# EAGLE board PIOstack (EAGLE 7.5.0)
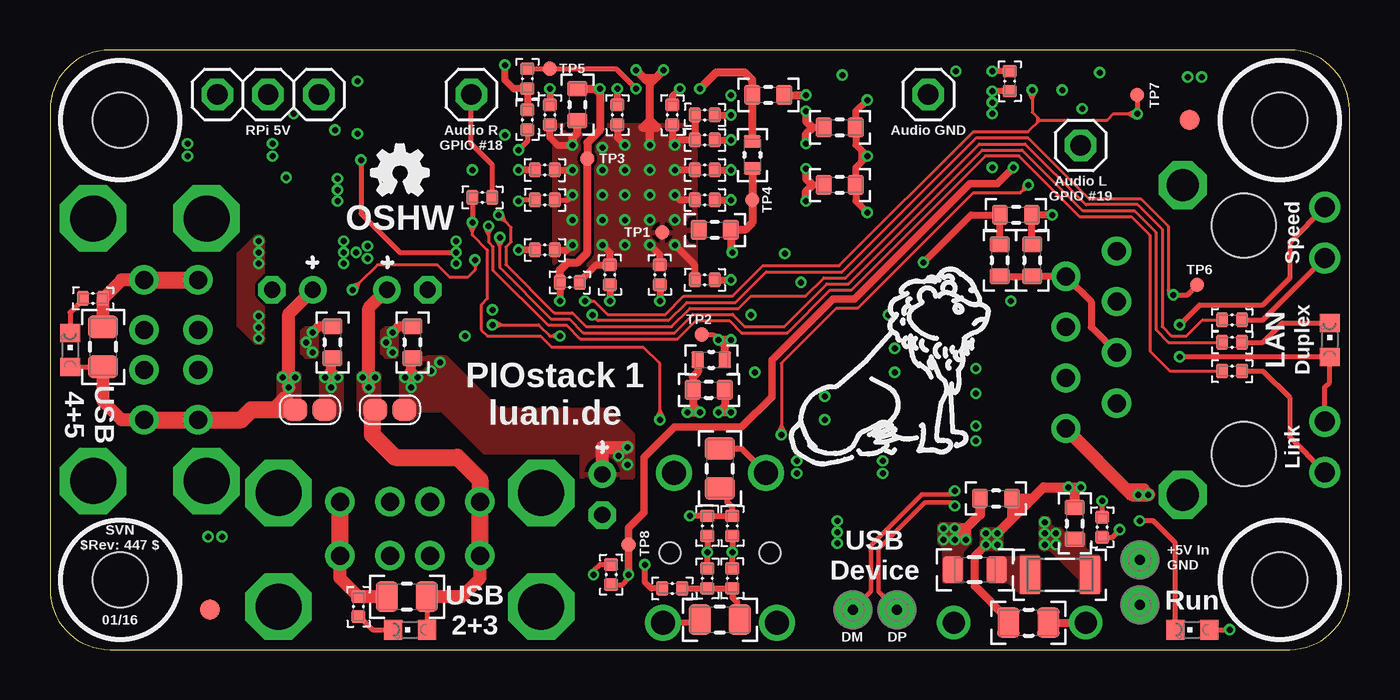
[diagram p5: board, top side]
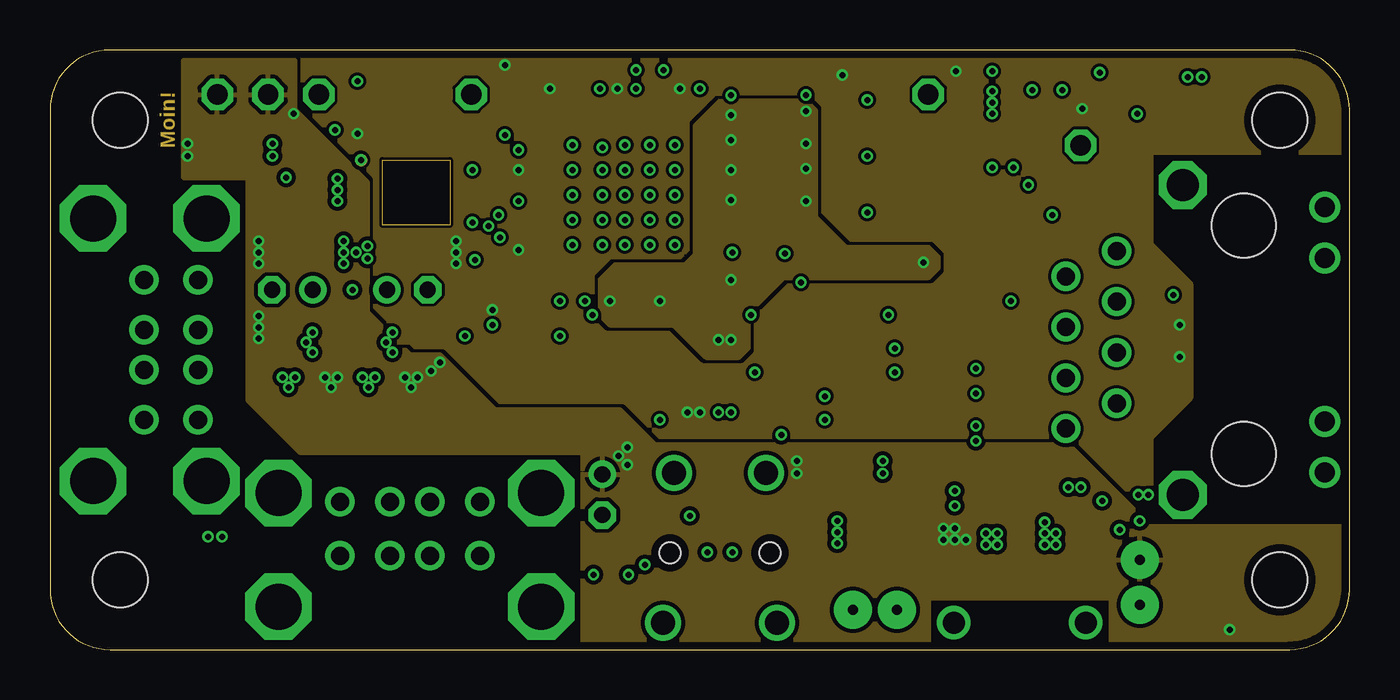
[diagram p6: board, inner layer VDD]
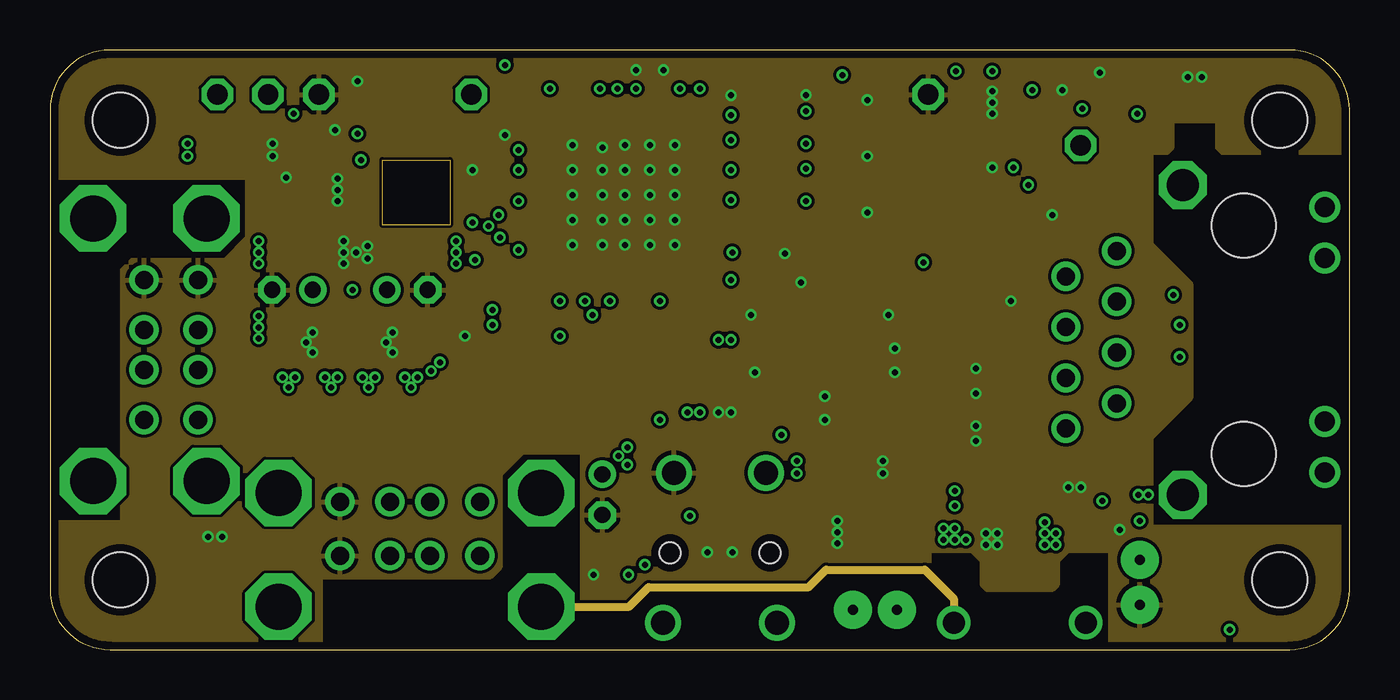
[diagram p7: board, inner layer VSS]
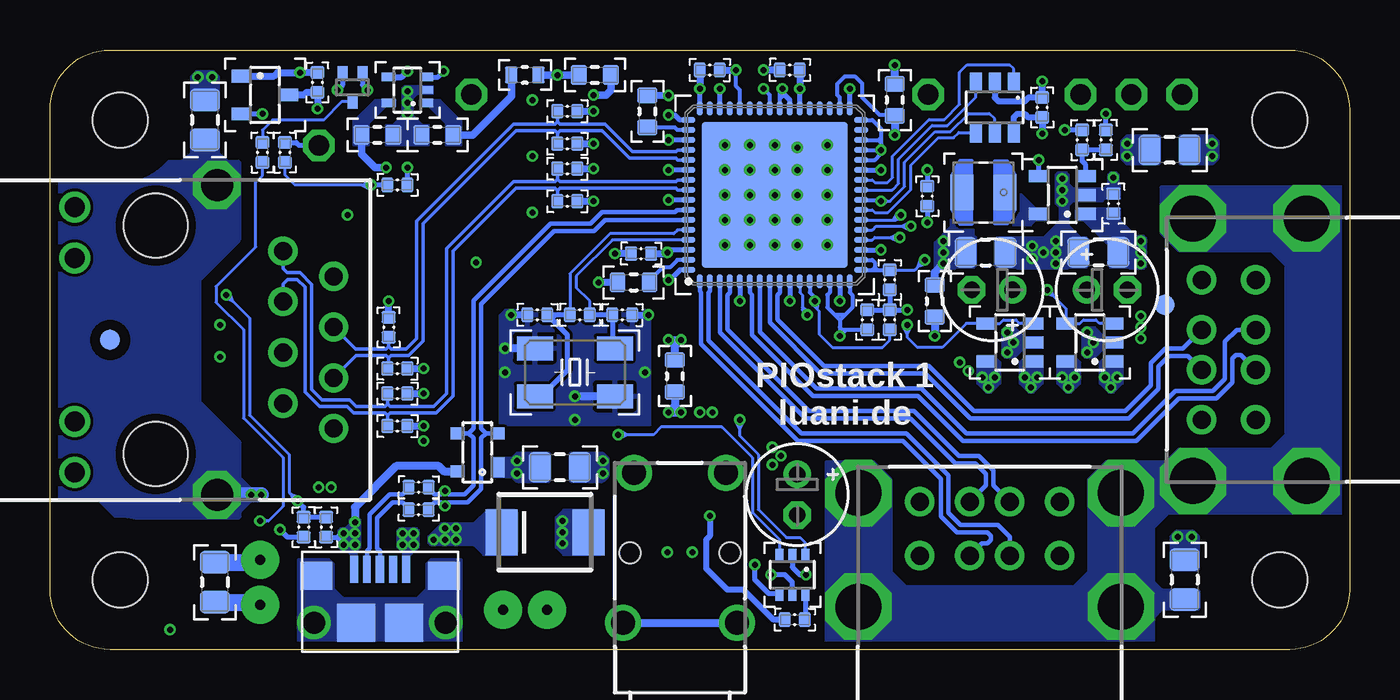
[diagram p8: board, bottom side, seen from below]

Size 65 x 30 mm. Coordinates in mm from the lower left corner, seen from the top.
Outline: 0,27 0,3 arc90 3,0 62,0 arc90 65,3 65,27 arc90 62,30 3,30 arc90 0,27
Copper layers (1+2*15+16): Top 0.035mm / dielectric 0.17mm / VDD 0.0175mm / dielectric 1.19mm / VSS 0.0175mm / dielectric 0.17mm / Bottom 0.035mm
Design rules "4-Layer 6x6-OSH *": minimum track width 6mil, minimum drill 0.3mm, track to track 6mil, track to pad 6mil, pad to pad 6mil, via to via 6mil, smd to smd 6mil, copper to edge 0.4mm, drill to drill 0.2mm, minimum pad ring 11mil, minimum via ring 5mil, stop-mask expansion 2.5mil, vias tented up to drill 0.5mm, thermal gap 8mil
Net classes: 1 USB-Diffpair: width 0.229 mm, clearance 0.508 mm to class 0, clearance 0.152 mm; 2 Ethernet-Diffpair: width 0.178 mm, clearance 0.762 mm to class 0, clearance 0.762 mm to class 1, clearance 0.152 mm; 3 Schirm: clearance 0.635 mm to class 0, clearance 0.635 mm to class 1, clearance 0.635 mm to class 2; 4 Takt: width 0.152 mm, clearance 0.508 mm to class 0, clearance 1.27 mm to class 1, clearance 1.27 mm to class 2; 5 Standardleiter neben Diffpair: clearance 0.508 mm to class 3, clearance 0.508 mm to class 4

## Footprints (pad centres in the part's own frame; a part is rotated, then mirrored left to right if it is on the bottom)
C-0603 = smd 0.8 x 1: 1 -0.8,0; 2 0.8,0
C-0402 = smd 0.6 x 0.7: 1 -0.5,0; 2 0.5,0
C-0805 = smd 1.1 x 1.5: 1 -1,0; 2 1,0
E2-5 = drill 0.813 pad 1.27: + -1.016,0 | drill 0.813 pad 1.27 octagon: - 1.016,0
BEL-1206 = smd 1 x 1.9: 1 -1.5,0; 2 1.5,0
HOLE_2.75R = hole 2.75: 0,0
QFN-64 = smd 0.69 x 0.28: 1 -4.325,3.75; 2 -4.325,3.25; 3 -4.325,2.75; 4 -4.325,2.25; 5 -4.325,1.75; 6 -4.325,1.25; 7 -4.325,0.75; 8 -4.325,0.25; 9 -4.325,-0.25; 10 -4.325,-0.75; 11 -4.325,-1.25; 12 -4.325,-1.75; 13 -4.325,-2.25; 14 -4.325,-2.75; 15 -4.325,-3.25; 16 -4.325,-3.75; 33 4.325,-3.75; 34 4.325,-3.25; 35 4.325,-2.75; 36 4.325,-2.25; 37 4.325,-1.75; 38 4.325,-1.25; 39 4.325,-0.75; 40 4.325,-0.25; 41 4.325,0.25; 42 4.325,0.75; 43 4.325,1.25; 44 4.325,1.75; 45 4.325,2.25; 46 4.325,2.75; 47 4.325,3.25; 48 4.325,3.75 | smd 0.28 x 0.69: 17 -3.75,-4.325; 18 -3.25,-4.325; 19 -2.75,-4.325; 20 -2.25,-4.325; 21 -1.75,-4.325; 22 -1.25,-4.325; 23 -0.75,-4.325; 24 -0.25,-4.325; 25 0.25,-4.325; 26 0.75,-4.325; 27 1.25,-4.325; 28 1.75,-4.325; 29 2.25,-4.325; 30 2.75,-4.325; 31 3.25,-4.325; 32 3.75,-4.325; 49 3.75,4.325; 50 3.25,4.325; 51 2.75,4.325; 52 2.25,4.325; 53 1.75,4.325; 54 1.25,4.325; 55 0.75,4.325; 56 0.25,4.325; 57 -0.25,4.325; 58 -0.75,4.325; 59 -1.25,4.325; 60 -1.75,4.325; 61 -2.25,4.325; 62 -2.75,4.325; 63 -3.25,4.325; 64 -3.75,4.325 | smd 7.3 x 7.3: PPAD 0,0
SOT23-6 = smd 0.6 x 1: 1 -0.95,-1.25; 2 0,-1.25; 3 0.95,-1.25; 4 0.95,1.25; 5 0,1.25; 6 -0.95,1.25
SOT-23/3 = smd 0.65 x 1: 1 -0.95,-1.175; 2 0.95,-1.175; 3 0,1.175
SOT-23/5 = smd 0.6 x 1: 1 -0.95,-1.175; 2 0,-1.175; 3 0.95,-1.175; 4 0.95,1.175; 5 -0.95,1.175
SOT-363/6 = smd 0.4 x 0.7: 1 -0.65,-0.95; 2 0,-0.95; 3 0.65,-0.95; 4 0.65,0.95; 5 0,0.95; 6 -0.65,0.95
SOT-353/5 = smd 0.4 x 0.7: 1 -0.65,-0.95; 2 0,-0.95; 3 0.65,-0.95; 4 0.65,0.95; 5 -0.65,0.95
JUMPER-2-R = smd 1.2 x 1.1: 1 -0.727,0; 2 0.727,0
BLM18P = smd 0.65 x 0.85: 1 -0.675,0; 2 0.675,0
MURATA_LQH3NP = smd 1.15 x 1.8: 1 -1.075,0; 2 1.075,0
BLM21P = smd 1 x 1.3: 1 -1.1,0; 2 1.1,0
CHIPLED-0603 = smd 0.9 x 1: A 0.85,0; C -0.85,0
FIDUCIAL-1MM/CREAM = smd 1 x 1: FIDUCIAL 0,0
ABRACON_ABM3B = smd 1.8 x 1.2: 1 -2,-1.2; 2 2,1.2; S@0 2,-1.2; S@1 -2,1.2
R-0402 = smd 0.6 x 0.7: 1 -0.5,0; 2 0.5,0
R-0603 = smd 0.8 x 1: 1 -0.8,0; 2 0.8,0
R-0805 = smd 1.1 x 1.5: 1 -1,0; 2 1,0
TESTPOINT-0906 = drill 0.5 pad 1.9: TP 0,0
SC75 = smd 0.5 x 0.7: 1 -0.5,-0.7; 2 0.5,-0.7; 3 0,0.7
TP07R = smd 0.7 x 0.7: TP 0,0
SOT143B = smd 1 x 0.7: 1 -0.75,-1 | smd 0.6 x 0.7: 2 0.95,-1; 3 0.95,1; 4 -0.95,1
DO214-AA = smd 1.6 x 2.3: A 2.175,0; K -2.175,0
BEL_SI-60062-F = drill 0.9: 1 -4.445,17.15; 2 -3.175,19.69; 3 -1.905,17.15; 4 -0.635,19.69; 5 0.635,17.15; 6 1.905,19.69; 7 3.175,17.15; 8 4.445,19.69 | drill 1: 9 -6.63,6.74; 10 -4.09,6.74; 11 4.09,6.74; 12 6.63,6.74 | drill 1.6 octagon: S@0 -7.75,13.85; S@1 7.75,13.85 | hole 3.2: -5.715,10.8; 5.715,10.8
KYCON_KUSBEX-ASFS2N = drill 0.9: B1 -3.5,12.55; B2 -1,12.55; B3 1,12.55; B4 3.5,12.55; T1 -3.5,15.25; T2 -1,15.25; T3 1,15.25; T4 3.5,15.25 | drill 2.3 octagon: S@0 -6.57,10; S@1 6.57,10; S@2 6.57,15.68; S@3 -6.57,15.68
FCI_10118193 = smd 0.4 x 1.35: 1 -1.3,4.125; 2 -0.65,4.125; 3 0,4.125; 4 0.65,4.125; 5 1.3,4.125 | drill 1.1: S@0 -3.3,1.45; S@1 3.3,1.45 | smd 1.9 x 1.9: S@2 -1.2,1.45; S@3 1.2,1.45 | smd 1.6 x 1.4: S@4 -3.2,3.8; S@5 3.2,3.8
1X01 = drill 1.016 octagon: 1 0,0
1X03 = drill 1.016 octagon: 1 -2.54,0; 2 0,0; 3 2.54,0
LUMBERG_1503-07 = drill 1.2: 1 2.3,11; 2@0 -2.85,3.5; 2@1 2.85,3.5; 3 -2.3,11 | hole 1.05: -2.5,7; 2.5,7

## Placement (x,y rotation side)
C201  4,7µ  [C-0603]  26.38,27.26 270 top
C202  4,7µ  [C-0603]  22.75,27.5 270 bottom
C203  100n  [C-0402]  28,29 180 bottom
C204  100n  [C-0402]  31.12,26.75 270 top
C205  100n  [C-0402]  26,18.38 0 top
C206  100n  [C-0402]  25,26.75 270 top
C207  100n  [C-0402]  28.38,26.75 270 top
C208  1µ  [C-0603]  35.92,27.75 0 top
C209  100n  [C-0402]  24.75,20 0 top
C210  100n  [C-0402]  32,29 0 bottom
C211  100n  [C-0402]  24.75,24 0 top
C212  1µ  [C-0603]  33.25,21 180 top
C213  100n  [C-0402]  35.44,19.81 180 bottom
C214  4,7µ  [C-0603]  33.75,13.69 270 bottom
C215  100n  [C-0402]  30.5,18.75 90 top
C216  100n  [C-0402]  28,18.75 90 top
C217  100n  [C-0402]  32.75,26.75 180 top
C218  100n  [C-0402]  32.75,25.5 180 top
C219  100n  [C-0402]  32.75,18.5 180 top
C220  100n  [C-0402]  32.75,24 180 top
C221  100n  [C-0402]  32.75,22.5 180 top
C222  100n  [C-0402]  15.38,27.12 90 bottom
C223  100n  [C-0402]  51.62,28.38 90 bottom
C224  18p  [C-0402]  36.38,16.75 0 bottom
C225  18p  [C-0402]  40.62,16.75 180 bottom
C301  1µF  [C-0603]  39.5,26.12 0 top
C302  1µF  [C-0603]  39.5,23.25 0 top
C303  1µF  [C-0603]  48.31,21.75 0 top
C304  15pF  [C-0402]  47.62,12.81 0 bottom
C305  15pF  [C-0402]  47.62,11.19 0 bottom
C306  15pF  [C-0402]  48.06,16.12 90 bottom
C307  15pF  [C-0402]  47.62,14.06 0 bottom
C308  22nF  [C-0603]  49.12,19.48 90 top
C401  1µ  [C-0603]  18.12,15.38 90 top
C402  1µ  [C-0603]  14.12,15.38 90 top
C403  100n  [C-0805]  48.94,1.35 0 top
C404  100n  [C-0805]  17.85,2.65 180 top
C405  47µ  [E2-5]  17.88,18 180 bottom
C406  100n  [C-0805]  2.65,15.15 90 top
C407  47µ  [E2-5]  12.12,18 0 bottom
C408  10n  [C-0603]  51.25,6.31 90 top
C409  100n  [C-0402]  52.62,6.12 270 top
C501  4,7µ  [C-0805]  12.56,19.88 180 bottom
C502  4,7µ  [C-0805]  9,25 180 bottom
C503  100n  [C-0402]  11.81,22.31 90 bottom
C504  4,7µ  [C-0805]  56.75,3.38 270 bottom
C505  10n  [C-0603]  47.31,7.56 0 top
C506  4,7µ  [C-0603]  32.95,13 0 top
C507  10µ  [C-0805]  18.2,19.88 0 bottom
C508  100n  [C-0402]  28.06,3.75 90 top
C509  100n  [C-0402]  34.12,3.56 90 top
C510  4,7µ  [C-0603]  20.75,17.44 270 bottom
C511  100n  [C-0402]  34.12,6.19 270 top
C512  47µ  [C-0805]  33.5,1.5 180 top
C513  47µ  [C-0805]  33.5,9.06 90 top
C514  100n  [C-0805]  39.5,9.12 180 bottom
C515  47µ  [E2-5]  27.62,7.75 270 bottom
C516  1µ  [C-0603]  37.75,28.75 0 bottom
C517  1µ  [C-0603]  45.62,25.75 180 bottom
C518  100n  [C-0402]  48,28.44 270 top
C519  4,7µ  [C-0603]  48.62,25.75 0 bottom
F501  2,5A  [BEL-1206]  50.5,3.75 180 top
H101  2.75mm  [HOLE_2.75R]  3.5,3.5 0 top
H102  2.75mm  [HOLE_2.75R]  61.5,3.5 0 top
H103  2.75mm  [HOLE_2.75R]  61.5,26.5 0 top
H104  2.75mm  [HOLE_2.75R]  3.5,26.5 0 top
IC201  LAN9514-JZX  [QFN-64]  28.75,22.75 90 bottom
IC202  93AA56AT-I/OT  [SOT23-6]  17.75,27.12 180 bottom
IC203  APX803-31SA  [SOT-23/3]  54.25,27.75 270 bottom
IC401  STMPS2171STR  [SOT-23/5]  17,15.38 90 bottom
IC402  STMPS2171STR  [SOT-23/5]  13,15.38 90 bottom
IC501  LM3671MF-3.3  [SOT-23/5]  14.38,22.75 90 bottom
IC502  74LVC2G17GW  [SOT-363/6]  27.88,3.75 180 bottom
IC503  AP7115-28SE  [SOT-353/5]  47.12,28 90 bottom
J401  X  [JUMPER-2-R]  17,12 180 top
J402  X  [JUMPER-2-R]  13,12 180 top
L201  BLM18PG121S  [BLM18P]  35.12,24.75 270 top
L202  BLM18PG121S  [BLM18P]  33.08,14.5 0 top
L501  2,2µH  [MURATA_LQH3NP]  18.31,22.88 180 bottom
L502  BLM21PG121S  [BLM21P]  46.25,4 180 top
L503  BLM18PG121S  [BLM18P]  41.25,28.75 180 bottom
LED201  grün  [CHIPLED-0603]  57.12,1 0 top
LED301  grün  [CHIPLED-0603]  64,15.5 270 top
LED401  grün  [CHIPLED-0603]  18,1 0 top
LED402  grün  [CHIPLED-0603]  1,15 270 top
LOGO1  LOGO-10MM-TPLACE  [10MM-TPLACE]  42,14.25 0 top
MARK101  FIDUCIAL-1.0/CREAM  [FIDUCIAL-1MM/CREAM]  8,2 0 top
MARK102  FIDUCIAL-1.0/CREAM  [FIDUCIAL-1MM/CREAM]  57,26.5 0 top
MARK103  FIDUCIAL-1.0/CREAM  [FIDUCIAL-1MM/CREAM]  62,15.5 270 bottom
MARK104  FIDUCIAL-1.0/CREAM  [FIDUCIAL-1MM/CREAM]  9.25,17.25 0 bottom
OSHW  OSHW-3MM-FILL-TPLACE  [OSHW-FILL-3MM-TPLACE]  17.5,24 0 top
Q201  25MHz  [ABRACON_ABM3B]  38.75,13.88 180 bottom
R201  10k  [R-0402]  23.88,26.5 90 top
R202  10k  [R-0402]  23,16.5 90 bottom
R203  10k  [R-0402]  24.75,22.5 180 top
R204  1M  [R-0402]  38.5,16.75 180 bottom
R205  360R  [R-0402]  54.38,24.88 270 bottom
R301  12,4k  [R-0603]  35.12,26.93 270 bottom
R302  10k  [R-0402]  23.88,28.56 270 top
R303  0R  [R-0805]  57.25,26.5 270 bottom
R304  360R  [R-0402]  59.12,15.38 0 top
R305  49,9  [R-0402]  39.12,24.06 0 bottom
R306  49,9  [R-0402]  39.12,22.44 0 bottom
R307  49,9  [R-0402]  39.12,26.94 0 bottom
R308  360R  [R-0402]  59.12,16.5 0 top
R309  49,9  [R-0402]  39.12,25.31 0 bottom
R310  360R  [R-0402]  59.12,13.94 0 top
R311  10R  [R-0603]  47.5,19.48 90 top
R401  12k  [R-0603]  35.81,18.38 0 bottom
R402  10k  [R-0402]  24.12,16.5 90 bottom
R403  1M  [R-0805]  8.25,3.5 270 bottom
R404  10k  [R-0402]  23,18.5 270 bottom
R405  360R  [R-0402]  15.43,2.15 270 top
R406  360R  [R-0402]  2.15,17.57 180 top
R407  0R  [R-0402]  46.56,8.12 180 bottom
R408  0R  [R-0402]  46.56,7 180 bottom
R409  10k  [R-0402]  52.31,6.12 90 bottom
R410  10k  [R-0402]  51.19,6.12 270 bottom
R501  1k  [R-0402]  12.19,25.5 90 bottom
R502  360R  [R-0402]  13.38,25.5 270 bottom
R503  100R  [R-0402]  53.25,24.88 270 bottom
R504  100R  [R-0402]  21.62,22.62 180 top
R505  470R  [R-0402]  47.62,23.25 180 bottom
R506  470R  [R-0402]  21.12,22.69 270 bottom
R507  100R  [R-0402]  31.12,3.06 0 top
R508  100R  [R-0402]  27.75,1.5 180 bottom
R509  100R  [R-0402]  32.88,3.56 270 top
R510  100R  [R-0402]  32.88,6.19 90 top
SP401  [TESTPOINT-0906]  54.5,4.5 0 top
SP402  [TESTPOINT-0906]  54.5,2.25 0 top
SP403  [TESTPOINT-0906]  42.35,2 0 top
SP404  [TESTPOINT-0906]  40.15,2 0 top
T201  DMG1012T  [SC75]  49.88,28.12 180 bottom
TP1  PTR1TP07R  [TP07R]  30.62,20.88 0 top
TP2  PTR1TP07R  [TP07R]  32.59,15.76 0 top
TP3  PTR1TP07R  [TP07R]  26.88,24.56 0 top
TP4  PTR1TP07R  [TP07R]  35.12,22.5 0 top
TP5  PTR1TP07R  [TP07R]  25,29.06 0 top
TP6  PTR1TP07R  [TP07R]  57.38,18.25 0 top
TP7  PTR1TP07R  [TP07R]  54.38,27.75 0 top
TP8  PTR1TP07R  [TP07R]  28.94,5.25 0 top
TVS401  PRTR5V0U2X  [SOT143B]  43.62,9.88 90 bottom
TVS501  SMBJ5V0A  [DO214-AA]  40.25,5.88 0 bottom
X301  SI-60062-F  [BEL_SI-60062-F]  70.5,15.5 270 bottom
X401  KUSBEX-ASFS2N  [KYCON_KUSBEX-ASFS2N]  18,-7.85 0 bottom
X402  KUSBEX-ASFS2N  [KYCON_KUSBEX-ASFS2N]  -7.85,15 90 bottom
X403  10118193-0001  [FCI_10118193]  48.5,-0.1 0 bottom
X501  Audio 1  [1X01]  51.55,25.23 0 top
X502  Audio 0  [1X01]  21.07,27.77 0 top
X503  Audio G  [1X01]  43.93,27.77 0 top
X504  RPi 5V  [1X03]  10.91,27.77 0 top
X505  1503_07  [LUMBERG_1503-07]  33.5,-2.15 0 bottom

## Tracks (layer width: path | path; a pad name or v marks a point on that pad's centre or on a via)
15KP/1
  VSS 0: 16.62,24.5 20,24.5 20,21.25 16.62,21.25 16.62,24.5
15KP/2
  VDD 0: 16.62,24.5 20,24.5 20,21.25 16.62,21.25 16.62,24.5
+3V3  (via drill 0.3)
  Top 0.254: X301.11 63.76,13.13 64,13.38 LED301.A v56.5,14.65 | X301.9 62,20.37 62,18.58 60.67,17.25 57.5,17.25 v56.5,16.25 | v15.55,24.5 15.55,21.82 17.5,19.88 v20.31,19.88
  Top 0.356: v31.5,28.06 31.12,27.69 C204.1 | C211.1 v23.44,24 | C207.1 v28.38,28.06 | C209.1 v23.44,20 | v25,28.06 C206.1 | R201.2 R302.2 23.19,28.06 22.75,28.5 v22.75,29.25
  Top 0.406: L202.1 32.4,13.9 32.15,13.65 C506.1 32.15,12.22 | 32.15,12.22 v32.5,11.88 v31.88,11.88 32.15,12.15 32.15,12.22
  Bottom 0.203: IC201.40 28.5,27.56 | 28.5,27.56 28.5,27.94 v28.38,28.06 | 28.19,27.69 28.38,27.69 28.5,27.56
  Bottom 0.254: IC201.33 v25,28.06 | IC201.27 v23.44,24 | IC201.19 v23.44,20 | IC201.46 v31.5,28.06 | IC201.39 28,27.5 28.19,27.69 28.38,27.88 v28.38,28.06 | R404.2 R202.2 | R402.2 R202.2 | R202.2 v22.12,17 | IC501.4 v15.55,24.5 | IC503.3 45.6,28.65 v45.31,28.94
  Bottom 0.305: C222.1 16.06,26.62 16.25,26.81 16.62,26.81 16.8,26.64 IC202.6
  Bottom 0.356: C222.1 v15.38,25.81 | v51.62,27.06 C223.1 52.19,27.88 52.31,27.75 IC203.3
  Bottom 0.381: L503.1 v39.62,28.75 C516.1
  Bottom 0.406: C202.1 v22.75,29.25 | C510.1 20.75,18.88 v20.31,19.31
  other vias: 20.31,20.44
  pour Bottom (rank 2, no thermals): 19.5,24.5 18.89,24.5 18.81,24.43 18.81,20.75 18.69,20.62 18.69,19.23 18.79,19.12 19.69,19.12 19.75,19.06 20.75,19.06 20.75,20.38 19.94,21.19 19.94,24.06
  pour VDD (rank 2, no thermals): 0,23.62 0,27 arc-90 3,30 62,30 arc-90 65,27 65,24.85 55.05,24.85 55.05,20.3 57.05,18.3 57.05,12.6 55.05,10.6 55.05,6.15 65,6.15 65,3 arc-90 62,0 53.05,0 53.05,2.6 43.95,2.6 43.95,0 26.62,0 26.62,9.88 9.88,9.88 9.88,23.62
+3V3_A  (via drill 0.3)
  Top 0.254: TP2.TP 33.17,15.76 v33.44,15.5
  Top 0.356: C218.1 v34.06,25.5 | C220.1 v34.06,24 | C221.1 v34.06,22.5 | C216.1 v28,17.44 | C215.1 v30.5,17.44 | C217.1 v34.06,26.75 | C219.1 v34.06,18.5 | C301.1 38.12,26.12 | C302.1 38.12,23.25 | R311.2 47.51,20.27 C303.1 46.06,21.75 v43.69,19.38
  Top 0.406: v37.81,26.94 37.81,26.44 38.12,26.12 37.81,25.81 v37.81,25.31 | v37.81,24.06 37.81,23.56 38.12,23.25 37.81,22.94 v37.81,22.44 | L202.2 33.75,15.19 | 33.75,15.19 v33.44,15.5 v34.06,15.5 33.75,15.19
  Bottom 0.254: IC201.10 v28,17.44 | IC201.5 v30.5,17.44 | IC201.57 v34.06,22.5 | IC201.54 v34.06,24 | IC201.51 v34.06,25.5 | IC201.64 33.5,19 34,18.5 v34.06,18.5 | IC201.49 33.5,26.5 33.75,26.75 v34.06,26.75
  Bottom 0.356: R307.2 v37.81,26.94 | R309.2 v37.81,25.31 | R305.2 v37.81,24.06 | R306.2 v37.81,22.44
  Bottom 0.406: C214.1 33.75,15.19 | 33.75,15.19 v33.44,15.5 v34.06,15.5 33.75,15.19
  pour VDD (no thermals): 34.94,15.12 34.94,16.88 36.69,18.62 43.94,18.62 44.44,19.12 44.44,19.62 43.94,20.12 39.81,20.12 38.31,21.62 38.31,26.94 37.81,27.44 33.5,27.44 32.25,26.19 32.25,19.75 31.75,19.25 28.25,19.25 27.5,18.5 27.5,16.75 28,16.25 31.19,16.25 32.81,14.62 34.44,14.62
+5V  (via drill 0.3)
  Top 0.254: LED201.A v59,1
  Top 0.508: 14.06,13.94 v13.75,13.62 v14.38,13.62 14.06,13.94 | 18.06,13.94 v17.75,13.62 v18.38,13.62 18.06,13.94 | C505.1 46.51,6.76 45.81,6.06 | 45.81,6.06 v45.25,5.5 | 45.81,6.06 45.56,6.06 | 45.81,6.06 45.81,5.81 | 14.06,13.94 14.06,14.57 C402.1 | 18.06,13.94 18.06,14.57 C401.1
  Top 0.65: C515.+ 27.62,10.12 v28.88,10.12
  Bottom 0.254: R501.2 v12.19,26.81
  Bottom 0.85: C504.1 54.62,4.38 SP401.TP
  other vias: 44.69,6.06 44.69,5.5 45.25,6.06 37.35,9.44 37.35,8.81 10.44,20.44 10.44,19.88 45.81,5.5 10.44,19.31 14.06,13.12 18.06,13.12 28.88,9.25 28.44,9.69 19.06,13.94 19.5,14.38 10.44,16.12 10.44,15.56 10.44,16.69 6.88,25.31 6.88,24.69
  pour Bottom (no thermals): 14.62,14.69 14.62,13.32 14.18,12.88 13.95,12.88 13.5,13.32 13.5,14.39 13.8,14.69
  pour Top (rank 2, no thermals): 44.69,5.06 44.69,3.38 45.62,3.38 45.62,4.88 46.06,5.31 46.06,5.72 45.48,6.31 44.54,6.31 44.44,6.21 44.44,5.31
  pour Bottom (rank 2, no thermals): 43.12,7 41.8,7 41.65,6.85 41.65,4.9 41.8,4.75 43.31,4.75 43.81,5.25 45.96,5.25 46.06,5.35 46.06,5.66 45.41,6.31 43.81,6.31
  pour Bottom (no thermals): 38.95,8.47 37.38,8.47 37.12,8.72 37.12,9.53 37.38,9.78 38.95,9.78
  pour Bottom (rank 2, no thermals): 13.31,21.5 13.61,21.5 13.69,21.57 13.69,21.99 13.61,22.06 11.5,22.06 11.5,21.5 10.69,20.69 10.29,20.69 10.19,20.59 10.19,19.16 10.29,19.06 11,19.06 11.06,19.12 11.96,19.12 12.06,19.23 12.06,20.25
  pour Bottom (no thermals): 18.62,14.69 18.62,13.32 18.18,12.88 17.95,12.88 17.5,13.32 17.5,14.39 17.8,14.69
  pour Top (no thermals): 14.62,12 14.62,13.78 14.53,13.88 13.6,13.88 13.5,13.78 13.5,11.5 14.12,11.5
  pour Top (no thermals): 18.62,12 18.62,13.78 18.52,13.88 17.6,13.88 17.5,13.78 17.5,11.5 18.12,11.5
  pour VDD (isolate 0.2): 26.62,0 43.95,0 43.95,2.6 53.05,2.6 53.05,0 62,0 arc90 65,3 65,6.15 55.05,6.15 50.95,10.25 30.25,10.25 28.5,12 22.25,12 19.5,14.75 18,14.75 15.88,16.88 15.88,23.38 12.25,27 12.25,29.48 6.67,29.48 6.67,23.62 9.88,23.62 9.88,12.5 12.5,9.88 26.62,9.88
  pour Top: 26.62,8.62 26.62,9.88 21.75,9.88 19.62,12 18.5,12 18.5,13.75 18.62,13.88 18.62,14.62 19.75,14.62 22.38,12 27.88,12 29.12,10.75 29.12,8.62
  pour Top: 10.69,20.59 10.69,15.41 10.59,15.31 10.25,15.31 9.38,16.19 9.38,19.81 10.25,20.69 10.59,20.69
  pour Bottom (no thermals): 8.45,24.35 6.88,24.35 6.62,24.6 6.62,25.4 6.88,25.65 8.45,25.65
+VB2-3  (via drill 0.3)
  Top 0.254: C404.1 LED401.A
  Top 0.5: v16.25,13.62 v15.62,13.62
  Top 0.65: X401.B1 21.5,3.58 20.57,2.65 C404.1 | v15.94,13.12 15.94,17.08 C405.+
  Top 0.85: X401.B1 X401.T1 21.5,8.5 20.38,9.62 17.25,9.62 16.12,10.75 16.12,12 J401.2
  pour Bottom (no thermals): 15.38,14.69 15.38,13.32 15.82,12.88 16.05,12.88 16.5,13.32 16.5,14.39 16.2,14.69
  pour Top (no thermals): 15.38,12 15.38,13.78 15.47,13.88 16.4,13.88 16.5,13.78 16.5,11.5 15.88,11.5
+VB4-5  (via drill 0.3)
  Top 0.254: LED402.A C406.1
  Top 0.5: v11.62,13.62 v12.25,13.62
  Top 0.65: X402.B1 3.58,11.5 2.65,12.43 C406.1 | v11.94,13.12 11.94,16.8 C407.+
  Top 0.85: X402.B1 X402.T1 9.56,11.5 10.06,12 11.25,12 | J402.2 11.25,12 | 11.25,12 11.75,12.5
  pour Bottom (no thermals): 11.38,14.69 11.38,13.32 11.82,12.88 12.05,12.88 12.5,13.32 12.5,14.39 12.2,14.69
  pour Top (no thermals): 11.38,12 11.38,13.78 11.47,13.88 12.4,13.88 12.5,13.78 12.5,11.5 11.88,11.5
AUD.PWM0
  Top 0.254: R504.1 22.12,24.25 21.07,25.3 X502.1
AUD.PWM1
  Bottom 0.254: R503.1 52.69,25.38 52.54,25.23 X501.1
ETH.AMDIX  (via drill 0.3)
  Top 0.254: R302.1 TP5.TP 28.31,29.06 v29.31,28.06
  Bottom 0.203: IC201.41 29,27.75 v29.31,28.06
ETH.L_FDX  (via drill 0.3)
  Top 0.152: 22.5,20.18 22.5,19.11 25.07,16.54 25.98,16.54 26.67,15.85 31.24,15.85 32.16,16.76 34.14,16.76 34.75,16.15 36.73,16.15 38.86,18.29 39.93,18.29 46.63,24.99 48.62,24.99 51.66,21.95 54.25,21.95 55.32,20.88 55.32,16 55.95,15.38 R304.1 | 22.5,20.18 22.5,20.25 | 22.5,20.25 v22.5,20.62 | v22.5,20.62 22.68,20.54 22.5,20.25 | 22.5,20.18 22.32,20.54 v22.5,20.62
  Bottom 0.152: IC201.20 23.88,20.5 23.75,20.62 22.95,20.62 | 22.95,20.62 v22.5,20.62 | 22.95,20.62 22.59,20.8 v22.5,20.62 | 22.95,20.62 22.59,20.45 v22.5,20.62
ETH.L_LNK  (via drill 0.3)
  Top 0.152: v21.94,21.19 21.94,20.74 | 21.94,20.74 21.94,20.38 22.17,20.14 22.17,18.97 24.92,16.23 25.83,16.23 26.52,15.54 31.39,15.54 32.31,16.46 33.98,16.46 34.59,15.85 36.88,15.85 39.01,17.98 40.08,17.98 46.79,24.69 48.46,24.69 51.51,21.64 54.1,21.64 55.02,20.73 55.02,14.94 56.01,13.94 R310.1 | 21.94,20.74 22.12,21.1 v21.94,21.19 | 21.94,20.74 21.76,21.1 v21.94,21.19
  Bottom 0.152: IC201.21 23.88,21 23.69,21.19 22.39,21.19 | 22.39,21.19 v21.94,21.19 | 22.39,21.19 22.03,21.37 v21.94,21.19 | 22.39,21.19 22.03,21.01 v21.94,21.19
ETH.L_SPD  (via drill 0.3)
  Top 0.152: R308.1 57.65,16.5 56.84,15.7 56.08,15.7 55.63,16.15 55.63,21.03 54.41,22.25 51.82,22.25 48.77,25.3 46.48,25.3 39.78,18.59 38.71,18.59 37.8,17.68 35.05,17.68 34.44,17.07 32,17.07 31.09,16.15 26.82,16.15 26.14,16.84 25.22,16.84 22.81,19.25 22.81,20.14 23.06,20.39 23.06,21.12 22.76,21.43 | 22.76,21.43 v22.44,21.75 | 22.76,21.43 22.63,21.81 v22.44,21.75 | 22.76,21.43 22.37,21.56 v22.44,21.75
  Bottom 0.152: IC201.22 22.81,21.5 | 22.81,21.5 22.69,21.5 v22.44,21.75 | 22.81,21.5 22.61,21.85 v22.44,21.75 | 22.81,21.5 22.41,21.55 v22.44,21.75
ETH.RD_N
  Bottom 0.178: IC201.53 33.6,24.5 33.69,24.59 36.01,24.59 37.38,25.96 39.5,25.96 39.62,25.84 | 48.06,14.59 47.94,14.71 47.06,14.71 46.34,15.43 46.34,21.31 41.68,25.96 39.75,25.96 39.62,25.84 | 48.06,14.59 48.19,14.71 49.7,14.71 X301.6 | R309.1 39.62,25.84 | 48.06,14.59 48.06,14.06 C307.1
ETH.RD_P
  Bottom 0.178: IC201.52 33.6,25 33.69,24.91 35.87,24.91 37.24,26.29 39.5,26.29 39.62,26.41 | 48.06,15.16 47.94,15.04 47.19,15.04 46.66,15.57 46.66,21.44 41.82,26.29 39.75,26.29 39.62,26.41 | 48.06,15.16 48.19,15.04 49.72,15.04 X301.4 | R307.1 39.62,26.41 | 48.06,15.16 C306.1
ETH.TD_N
  Bottom 0.178: IC201.56 33.6,23 33.69,23.09 39.5,23.09 39.62,22.96 | 48.12,11.71 48,11.84 45.68,11.84 44.84,12.68 44.84,19.93 41.68,23.09 39.75,23.09 39.62,22.96 | 48.12,11.71 48.25,11.84 49.82,11.84 50.14,12.16 51.52,12.16 52.24,12.89 52.24,18.14 52.63,18.52 53.12,18.52 53.35,18.3 X301.3 | R306.1 39.62,22.96 | C305.1 48.12,11.71
ETH.TD_P
  Bottom 0.178: IC201.55 33.6,23.5 33.69,23.41 39.5,23.41 39.62,23.54 | 48.12,12.29 48,12.16 45.82,12.16 45.16,12.82 45.16,20.07 41.82,23.41 39.75,23.41 39.62,23.54 | 48.12,12.29 48.25,12.16 49.68,12.16 50.01,12.49 51.38,12.49 51.91,13.02 51.91,18.27 52.49,18.85 53.15,18.85 53.35,19.05 X301.1 | R305.1 39.62,23.54 | C304.1 48.12,12.29
ETH.TR-CT
  Top 0.356: X301.5 52.08,16.14 52.08,17.41 X301.2 C308.1 R311.1
GND  (via drill 0.3)
  Top 0.254: R203.1 25.88,22.5 v26.12,22.75 | C409.2 53.12,5.62 v53.5,6 | C508.2 27.5,4.25 27.19,3.94 v27.19,3.75
  Top 0.305: C518.2 v47.12,27.94 | R509.1 v32.88,4.88 R510.1 | C509.2 v34.12,4.88 C511.2
  Top 0.356: C217.2 C218.2 31.5,25.5 v31.25,25.25 31.12,25.38 C204.2 | C215.2 30.5,19.75 v30,20.25 | v27.62,20.25 28,19.88 C216.2 27.31,19.25 26.5,18.44 C205.2 | C209.2 25.88,20 v26.12,20.25 | C211.2 v26.12,24 | C220.2 v31.25,24 | C221.2 31.5,22.5 v31.25,22.75 | C207.2 28.38,25.62 v28.75,25.25 | v26.12,25.25 25.38,25.25 25,25.62 C206.2 | C219.2 32.25,19.25 v31.25,20.25 | 40.58,24.98 40.3,25.26 C301.2 40.3,26.93 v40.88,27.5 | 40.58,24.98 v40.88,24.69 40.3,24.11 C302.2 40.3,22.45 v40.88,21.88 | v50.12,21.75 C303.2 C308.2 | 40.58,24.98 40.58,24.42
  Top 0.406: C201.2 26.38,25.88 26.12,25.62 v26.12,25.25 | C208.2 v37.81,27.75 | C506.2 33.75,12.19 | 33.75,12.19 v33.44,11.88 v34.06,11.88 33.75,12.19 | v46.81,5.25 46.25,4.69 46.25,3.19 47.94,1.5 C403.1 | v30,25.25 30,26.5 | 30,26.5 30,28.31 | 30,28.31 30.31,28.62 | 30.31,28.62 v30.69,29 | v29.31,29 29.69,28.62 | 29.69,28.62 30,28.31 | 30,26.5 29.62,26.12 30.38,26.12 30,26.5 | 29.69,28.62 30.31,28.62
  Top 0.508: v50.94,8.12 v51.56,8.12 51.25,7.81 | C408.2 51.25,7.81 | 51.25,7.81 v50.94,8.12 | 49.12,7.56 C505.2 48.11,6.55 | 49.12,7.56 49.69,8.12 v50.94,8.12 | 48.11,6.55 v47.38,5.81 | 48.11,6.55 49.12,7.56 | C402.2 13.43,16.18 v13.12,15.88 | C401.2 17.43,16.18 v17.12,15.88
  Top 0.65: C406.2 R406.1 3.58,18.5 X402.B4 | C404.2 R405.1 14.5,3.58 X401.B4
  Top 0.85: X402.B4 X402.T4 | X401.B4 X401.T4
  Bottom 0.203: IC201.44 30.5,28 30.69,28.19 v30.69,29 | IC201.34 25.5,27.62 25.62,27.75 25.62,28.31 25.25,28.69 24.75,28.69 24.38,28.31 24.38,27.62 23.5,26.75 22.75,26.75 C202.2
  Bottom 0.254: R409.1 53.12,5.62 v53.5,6 | T201.2 50.38,28.25 v50.62,28 | v21.12,24 R506.1 | R505.1 v47.12,24.12 | R502.1 v14.25,26 | IC502.2 27.88,4.12 27.5,3.75 v27.19,3.75
  Bottom 0.305: C222.2 16.06,27.62 16.25,27.44 17.56,27.44 17.75,27.62 IC202.2
  Bottom 0.356: C213.2 v36.75,19.81 | C210.2 v30.69,29 | C203.2 v29.31,29 | C306.2 v48.06,17.44 | C307.2 v46.31,14.06 | C304.2 v46.31,12.81 | C305.2 v46.31,11.19 | R301.1 v34.06,27.73 | R401.1 v37.56,18.38 | C225.2 v41.94,16.75 | C224.2 v35.06,16.75 | C222.2 v15.38,28.44 | C223.2 v52.5,28.88 53.62,28.88 53.8,28.7 IC203.1
  Bottom 0.381: C516.2 36.95,27.99 37.19,27.75 v37.81,27.75
  Bottom 0.406: C202.2 v22.75,25.75 | Q201.S@1 v38.75,12.68 | Q201.S@0 v42.25,15.07 | C214.2 33.75,12.19 | 33.75,12.19 v33.44,11.88 v34.06,11.88 33.75,12.19 | C510.2 v20.75,15.69
  Bottom 0.85: C504.2 54.62,2.38 SP402.TP
  other vias: 28.75,22.75 30,21.5 28.75,20.25 27.62,21.5 30,24 27.62,24 57.6,28.65 56.9,28.65 27.62,25.12 26.12,21.5 28.75,24 27.62,22.75 30,22.75 28.75,21.5 31.25,21.5 14.38,23 14.38,23.56 14.38,22.44 14.69,19.88 14.69,19.31 46.81,5.81 47.38,5.25 39.38,6.44 39.38,5.88 8.6,5.65 7.9,5.65 13.12,14.88 17.12,14.88 41.65,8.81 39.38,5.31 38.75,11.5 42.25,13.88 41.65,9.44 14.69,20.44 35.25,13.88 12.81,15.38 16.81,15.38 15.31,19.88 15.88,20.19 11.81,23.62 11.12,25.31 11.12,24.69 47.12,27.38 15.88,19.56 47.12,26.81 46.31,10.44
  pour Top: 25.25,26.25 32.25,26.25 32.25,19.25 25.25,19.25
  pour Bottom (rank 2, no thermals): 56.6,27.05 56.6,28.62 56.85,28.88 57.65,28.88 57.9,28.62 57.9,27.05
  pour VSS (rank 2): 3,30 62,30 arc-90 65,27 65,24.85 58.65,24.85 58.4,25.1 58.4,26.45 56.1,26.45 56.1,25.1 55.85,24.85 55.05,24.85 55.05,20.3 57.05,18.3 57.05,12.6 55.05,10.6 55.05,6.15 65,6.15 65,3 arc-90 62,0 53.05,0 53.05,4.95 50.88,4.95 50.38,4.45 50.38,3.25 50.12,3 46.88,3 46.62,3.25 46.62,4.45 46.12,4.95 43.95,4.95 43.95,0 26.62,0 26.62,9.88 23.6,9.88 22.5,8.78 22.5,4.12 22,3.62 13.5,3.62 13.5,0 3,0 arc-90 0,3 0,6.38 3.62,6.38 3.62,19 4.12,19.5 8.78,19.5 9.88,20.6 9.88,23.62 0,23.62 0,27 arc-90
  pour Bottom (no thermals): 7.6,4.05 7.6,5.62 7.85,5.88 8.65,5.88 8.9,5.62 8.9,4.05
  pour Bottom (rank 2, no thermals): 11.38,15.62 12.25,15.62 12.75,16.12 13.25,16.12 13.38,16 13.38,14.75 13.25,14.62 12.75,14.62 12.25,15.12 11.38,15.12
  pour Bottom (rank 2, no thermals): 15.38,15.62 16.25,15.62 16.75,16.12 17.25,16.12 17.38,16 17.38,14.75 17.25,14.62 16.75,14.62 16.25,15.12 15.38,15.12
  pour Bottom (rank 3, no thermals): 47.13,3.41 47.27,3.41 47.34,3.48 47.34,4.84 47.62,5.12 47.62,5.96 47.52,6.06 46.66,6.06 46.56,5.96 46.56,5.12 47.06,4.63 47.06,3.48
  pour Bottom (no thermals): 39.31,4.75 37.46,4.75 37.31,4.9 37.31,6.85 37.46,7 39.31,7 39.69,6.62 39.69,5.12
  pour Bottom: 35,11.25 42.5,11.25 42.5,16.75 42.25,17 35.25,17 35,16.75
  pour Bottom (no thermals): 40.05,9.78 41.62,9.78 41.88,9.53 42.88,9.53 42.88,8.72 41.88,8.72 41.62,8.47 40.05,8.47
  pour Top (rank 3): 47.62,6.06 47.62,5.1 47.52,5 46.56,5 46.56,5.96 46.66,6.06
  pour Bottom (rank 3, no thermals): 11.66,23.88 11.96,23.88 12.06,23.77 12.06,23.31 12.31,23.06 13.81,23.06 14.06,23.31 14.06,23.77 14.16,23.88 14.59,23.88 14.69,23.77 14.69,22.31 14.5,22.12 14.5,21.44 15.31,20.62 17.65,20.62 17.75,20.52 17.75,19.23 17.65,19.12 16.69,19.12 16.62,19.06 14.12,19.06 14.06,19.12 13.16,19.12 13.06,19.23 13.06,20.52 13.16,20.62 13.44,20.62 14.06,21.25 14.06,22.19 13.81,22.44 12.38,22.44 12.25,22.56 11.5,22.56 11.5,23.25 11.56,23.31 11.56,23.77
  pour Bottom (rank 2, no thermals): 45.88,28.19 47.27,28.19 47.38,28.09 47.38,26.75 47.88,26.25 48.19,26.25 48.19,25.25 46.06,25.25 46.06,26.25 46.38,26.25 46.88,26.75 46.88,27.56 46.62,27.81 45.88,27.81
  pour Top (no thermals): 12.56,14.81 12.75,14.62 13.28,14.62 13.38,14.72 13.38,16.02 13.28,16.12 12.75,16.12 12.56,15.94
  pour Top (no thermals): 16.56,14.81 16.75,14.62 17.27,14.62 17.38,14.72 17.38,16.02 17.27,16.12 16.75,16.12 16.56,15.94
  pour Bottom (no thermals): 9.55,25.65 11.12,25.65 11.38,25.4 11.38,24.6 11.12,24.35 9.55,24.35
GNDI
  Top 0.406: C403.2 X403.S@0
  VSS 0.406: X401.S@0 28.96,2.15 29.94,3.12 37.94,3.12 38.81,4 43.75,4 45.2,2.55 X403.S@1
  pour Bottom (no thermals): 26.12,9.38 23.88,9.38 23,8.5 23,3.88 22.25,3.12 13.75,3.12 13,3.88 13,8.5 12.12,9.38 9.12,9.38 8.5,10 3.88,10 3.12,10.75 3.12,19.25 3.88,20 8.5,20 9.38,20.88 9.38,23.12 0,23.12 0,6.88 9.12,6.88 9.88,6.12 9.88,3.38 9.44,2.94 7.6,2.94 7.6,2.06 9.44,2.06 9.88,1.62 9.88,0 26.12,0
  pour Bottom (no thermals): 44.45,0 44.45,4.45 45.92,4.45 46.12,4.25 46.12,3 46.62,2.5 50.38,2.5 50.88,3 50.88,4.25 51.08,4.45 52.55,4.45 52.55,0
GNDIO  (via drill 0.3)
  Top 0.65: 53.88,8 54.69,8 v54.94,7.75 v54.43,7.75 54.12,7.75 X301.8
  Bottom 0.75: v54.43,7.75 v54.94,7.75 X301.S@1
  pour Bottom (no thermals): 65,7.65 62.65,7.65 61.65,6.65 55.55,6.65 55.55,6.95 55,7.5 55,8 55.55,8.55 55.55,10.35 57.55,12.35 57.55,18.55 55.55,20.55 55.55,24.35 56.15,24.35 56.6,24.8 56.6,25.95 57.9,25.95 57.9,24.8 58.35,24.35 61.65,24.35 62.65,23.35 65,23.35
IC501.SW
  pour Bottom (no thermals): 15.06,21.96 15.06,21.6 15.16,21.5 15.69,21.5 15.94,21.25 17.74,21.25 17.81,21.32 17.81,24.43 17.74,24.5 17.12,24.5 16.69,24.06 16.69,23.06 15.69,22.06 15.16,22.06
IC503.BP  (via drill 0.3)
  Top 0.305: C518.1 v47.12,28.94
  Bottom 0.305: IC503.4 47.41,28.65 v47.12,28.94
IC503.VIN
  Bottom 0.381: C517.1 43.88,25.75 41.92,27.7 L503.2
  pour Bottom (no thermals): 45.19,25.25 45.19,26.31 46.06,27.19 46.5,27.19 46.5,27.5 45.5,27.5 44.44,26.44 44.44,25.25
N$1
  Top 0.254: X301.10 60.67,16.5 R308.2
N$2
  Bottom 0.203: IC201.50 33.62,26 33.75,26.12 R301.2
N$3
  Bottom 0.203: IC201.63 33.62,19.5 34,19.12 34.38,19.12 35.01,18.49 R401.2
N$4
  Bottom 0.254: R501.1 R502.2 13.38,24.44 13.2,24.26 IC501.3
N$6  (via drill 0.3)
  Top 0.254: LED201.C 56.27,5.35 55.19,6.44 v54.5,6.44
  Bottom 0.152: R205.2 54.38,23.72 54.71,23.39 54.71,20.14 56.69,18.16 56.69,17.37 55.32,16 55.32,11.58 53.34,9.6 53.34,7.16 54.06,6.44 54.19,6.44 | 54.19,6.44 v54.5,6.44 | v54.5,6.44 54.4,6.26 54.19,6.44 | v54.5,6.44 54.42,6.62 54.19,6.44
N$7
  Bottom 0.152: R205.1 54.38,26 53.88,26.5 51.31,26.5 50.39,27.43 T201.3
N$9
  Top 0.305: R507.2 R509.2 C509.1 34.12,2.62 34.38,2.38 34.38,1.5 C512.1
N$10
  Top 0.254: R406.2 1.65,17.52 1,16.88 LED402.C
N$11
  pour Top (no thermals): 47.94,3.38 46.98,3.38 46.88,3.48 46.88,4.53 46.98,4.62 48.5,4.62 48.56,4.69 49.4,4.69 49.5,4.59 49.5,2.91 49.4,2.81 48.56,2.81
N$12
  Top 0.254: X301.12 62,10.63 62,12.61 60.67,13.94 R310.2
N$13
  Top 0.254: R405.2 15.47,1.65 16.12,1 LED401.C
N$14
  Top 0.254: R304.2 60.67,15.38 61.65,16.35 LED301.C
N$15  (via drill 0.3)
  Top 0.305: v32,6.69 R510.2 C511.1 34.12,7.12 33.88,7.38 33.88,8.06 C513.1
  Bottom 0.305: v32,6.69 32,5.69 32.19,5.5 32.19,4.06 31.12,3 30.31,3 28.81,1.5 R508.2
N$16
  Top 0.305: 32.5,1.35 X505.2@1
  Top 0.356: C512.2 32.5,1.35
  Bottom 0.406: X505.2@0 X505.2@1
N$17
  Top 0.305: C513.2 34.59,10.06 X505.3
N$18  (via drill 0.3)
  Top 0.305: R507.1 30.06,3.06 29.75,3.38 v29.75,4.25
  Bottom 0.254: IC502.4 29.05,2.8 29.75,3.5 v29.75,4.25
N$19
  Bottom 0.254: IC502.6 27.23,1.5 R508.1
N$20  (via drill 0.3)
  Top 0.152: 48.68,22.99 48.55,22.86 46.18,22.86 40.39,17.07 39.32,17.07 36.58,14.33 36.58,11.2 | 48.68,22.99 v48.94,23.25 | 36.58,11.2 v36.58,10.75 | 48.68,22.99 49,23.06 v48.94,23.25 | 48.68,22.99 48.75,23.31 v48.94,23.25 | 36.58,11.2 36.4,10.84 v36.58,10.75 | 36.58,11.2 36.76,10.84 v36.58,10.75
  Bottom 0.152: v48.94,23.25 49.39,23.25 | 49.39,23.25 52.75,23.25 53.25,23.75 R503.2 | IC502.3 28.52,5.51 29.87,6.86 29.87,9.6 31.39,11.12 34.44,11.12 34.82,10.75 36.13,10.75 | 36.13,10.75 v36.58,10.75 | 49.39,23.25 49.03,23.43 v48.94,23.25 | 49.39,23.25 49.03,23.07 v48.94,23.25 | 36.13,10.75 36.49,10.57 v36.58,10.75 | 36.13,10.75 36.49,10.93 v36.58,10.75
  Bottom 0.254: R505.2 v48.94,23.25
N$21  (via drill 0.3)
  Top 0.152: 21.12,20.93 21.12,20.73 21.87,19.99 21.87,17.56 21.56,17.25 21.56,16 21.88,15.69 24.55,15.69 25.11,15.12 29.68,15.12 30.5,14.31 30.5,11.95 | 21.12,20.93 v21.12,21.38 | v30.5,11.5 30.5,11.95 | 21.12,20.93 21.3,21.29 v21.12,21.38 | 21.12,20.93 20.95,21.29 v21.12,21.38 | 30.5,11.95 30.32,11.59 v30.5,11.5 | 30.5,11.95 30.68,11.59 v30.5,11.5
  Top 0.254: R504.2 v21.12,21.38
  Bottom 0.152: IC502.1 27.23,5.35 27.49,5.61 28.17,5.61 29.57,7.01 29.57,9.75 30.5,10.69 30.5,11.05 | 30.5,11.05 v30.5,11.5 | 30.5,11.05 30.68,11.41 v30.5,11.5 | 30.5,11.05 30.32,11.41 v30.5,11.5
  Bottom 0.254: R506.2 v21.12,21.38
PHY.!RES  (via drill 0.3)
  Top 0.152: v26.75,17.44 27.07,17.44 | 27.07,17.44 27.22,17.44 27.89,16.76 30.79,16.76 31.7,17.68 34.14,17.68 35.66,19.2 39.47,19.2 46.18,25.91 48.92,25.91 49.51,26.5 | v49.12,28 49.12,27.55 | 49.12,27.55 49.12,26.89 49.39,26.62 | 49.39,26.62 49.51,26.5 | 49.39,26.62 49.39,26.43 | 49.51,26.5 52.88,26.5 53.17,26.8 53.92,26.8 | 53.92,26.8 v54.38,26.8 | 27.07,17.44 26.84,17.62 v26.75,17.44 | 27.07,17.44 26.84,17.26 v26.75,17.44 | 53.92,26.8 54.28,26.62 v54.38,26.8 | 53.92,26.8 54.28,26.98 v54.38,26.8 | 49.12,27.55 49.3,27.91 v49.12,28 | 49.12,27.55 48.95,27.91 v49.12,28
  Top 0.254: TP7.TP v54.38,26.8
  Bottom 0.152: R202.1 23,15.5 23.38,15.12 25.87,15.12 26.52,15.77 26.52,16.92 26.61,17.01 | v26.75,17.44 26.75,17.15 26.67,17.07 | 26.67,17.07 26.61,17.01 | 26.67,17.07 26.67,17.22 26.75,17.3 | 26.61,17.01 26.89,17.3 v26.75,17.44 | 26.61,17.01 26.55,17.41 v26.75,17.44
  Bottom 0.203: IC201.12 27,17.88 26.75,17.62 v26.75,17.44
  Bottom 0.254: IC203.2 v54.38,26.8 | T201.1 49.38,28.25 v49.12,28
PHY.EECLK
  Bottom 0.152: IC201.23 23.88,22 23.75,21.88 23.08,21.88 21.95,23.01 21.95,24.23 20.57,25.6 19.81,25.6 19.54,25.88 IC202.4
PHY.EECS  (via drill 0.3)
  Top 0.254: R203.2 23.5,22.5 v23.44,22.44
  Bottom 0.152: v23.44,22.44 23.11,22.44 | 23.11,22.44 22.98,22.44 22.25,23.16 22.25,24.38 20.73,25.91 19.96,25.91 19.05,26.82 18.02,26.82 17.75,26.55 IC202.5 | 23.11,22.44 23.35,22.26 v23.44,22.44 | 23.11,22.44 23.35,22.62 v23.44,22.44
  Bottom 0.203: IC201.24 23.5,22.5 v23.44,22.44
PHY.EEDI
  Bottom 0.152: IC201.26 23.88,23.5 23.75,23.38 23.11,23.38 22.86,23.62 22.86,24.69 21.03,26.52 20.27,26.52 19.51,27.28 19.51,28.88 19.13,29.26 17.01,29.26 16.8,29.05 IC202.1
PHY.EEDO
  Bottom 0.152: IC201.25 22.87,23 22.55,23.32 22.55,24.54 20.88,26.21 20.12,26.21 18.7,27.63 IC202.3
PHY.JTAG-PU  (via drill 0.3)
  Top 0.254: R201.1 23.88,25.44 v23.44,25
  Bottom 0.203: 23.44,25.5 23.44,25.38 | 23.44,25.38 v23.44,25 | IC201.29 v23.44,25 | IC201.30 23.56,25.5 | 23.56,25.5 23.44,25.5 | IC201.28 23.75,24.5 23.44,24.81 v23.44,25 | IC201.32 23.88,26.5 23.44,26.06 23.44,25.62 | 23.44,25.62 23.44,25.5 | 23.56,25.5 23.44,25.62 | 23.56,25.5 23.44,25.38
PHY.XI
  Bottom 0.152: IC201.61 36.88,20.5 38.69,18.69 38.69,18.12 38,17.44 R204.1
  Bottom 0.254: R204.1 C224.1 36.88,15.07 Q201.1
PHY.XO
  Bottom 0.152: IC201.60 33.62,21 33.81,20.81 37,20.81 39,18.81 R204.2
  Bottom 0.254: R204.2 39.75,16.75 | 39.75,16.75 C225.1 | C225.1 40.12,16.69 | Q201.2 40.45,12.68 39.12,14 39.12,15.75 39.88,16.5 | 39.88,16.5 C225.1 | 39.75,16.75 39.88,16.62 39.88,16.5
USB.D0_N  (via drill 0.3)
  Top 0.229: v45.25,7.94 45.07,7.75 43.61,7.75 41.06,5.2 41.06,2.91 SP404.TP
  Bottom 0.229: IC201.58 33.63,22 33.75,21.88 37.39,21.88 37.95,21.32 39.95,21.32 43.82,17.45 43.82,11.06 44.05,10.82 | TVS401.3 44.05,10.82 | R407.1 46.06,8.06 45.75,7.75 45.43,7.75 v45.25,7.94 45.07,7.75 44.27,7.75 43.82,8.2 43.82,10.59 44.05,10.82
USB.D0_P  (via drill 0.3)
  Top 0.229: v45.25,7.19 45.07,7.37 43.77,7.37 41.44,5.05 41.44,2.91 SP403.TP
  Bottom 0.229: IC201.59 37.23,21.5 37.8,20.93 39.8,20.93 43.43,17.3 43.43,11.06 43.2,10.82 | TVS401.2 43.2,10.82 | R408.1 46.06,7.06 45.75,7.37 45.43,7.37 v45.25,7.19 45.07,7.37 44.11,7.37 43.43,8.05 43.43,10.59 43.2,10.82
USB.D2_N
  Bottom 0.229: IC201.1 32.5,17.93 32.44,17.88 32.44,15.3 27.58,10.43 22.33,10.43 20.44,8.55 20.44,6.67 19.63,5.86 18.11,5.86 17.94,5.68 17.94,5.49 18.11,5.31 18.39,5.31 X401.B2
USB.D2_P
  Bottom 0.229: IC201.2 32,17.93 32.06,17.88 32.06,15.45 27.42,10.82 22.17,10.82 20.06,8.7 20.06,6.83 19.47,6.24 17.6,6.24 17,5.64 X401.B3
USB.D3_N
  Bottom 0.229: IC201.3 31.5,15.86 27.2,11.56 21.95,11.56 19.7,9.31 18.7,9.31 18.19,8.8 18.19,8.21 X401.T2
USB.D3_P
  Bottom 0.229: IC201.4 31,17.87 31.12,17.75 31.12,16.01 27.05,11.94 21.8,11.94 19.55,9.69 18.55,9.69 17.81,8.95 17.81,8.21 X401.T3
USB.D4_N
  Bottom 0.229: IC201.6 30,17.87 29.88,17.75 29.88,15.74 26.83,12.68 21.58,12.68 19.33,10.43 10.67,10.43 8.55,12.56 6.67,12.56 5.86,13.37 5.86,14.57 5.68,14.75 5.45,14.75 X402.B2
USB.D4_P
  Bottom 0.229: IC201.7 29.5,15.89 26.67,13.07 21.42,13.07 19.17,10.82 10.83,10.82 8.7,12.94 6.83,12.94 6.24,13.53 6.24,15.4 5.64,16 X402.B3
USB.D5_N
  Bottom 0.229: IC201.8 29,16.36 26.45,13.81 21.2,13.81 18.95,11.56 11.05,11.56 9.56,13.05 9.56,14.17 9.05,14.68 8.09,14.68 X402.T2
USB.D5_P
  Bottom 0.229: IC201.9 28.5,17.87 28.62,17.75 28.62,16.51 26.3,14.19 21.05,14.19 18.8,11.94 11.2,11.94 9.94,13.2 9.94,14.33 9.2,15.07 8.34,15.07 X402.T3
USB.EXT-DO_N
  Bottom 0.229: X403.2 49.15,4.94 49.02,5.07 49.02,6.75 48.02,7.75 47.37,7.75 47.06,8.06 R407.2
USB.EXT-DO_P
  Bottom 0.229: X403.3 48.5,4.94 48.63,5.07 48.63,6.6 47.86,7.37 47.37,7.37 47.06,7.06 R408.2
USB.PRTCTL2-3  (via drill 0.3)
  Top 0.152: v22.12,16.25 22.57,16.25 | 22.57,16.25 24.44,16.25 25,15.69 25.18,15.69 | 25.18,15.69 v25.5,15.69 | 25.18,15.69 25.41,15.51 v25.5,15.69 | 25.18,15.69 25.41,15.87 v25.5,15.69 | 22.57,16.25 22.21,16.43 v22.12,16.25 | 22.57,16.25 22.21,16.07 v22.12,16.25
  Bottom 0.152: IC401.3 16.51,16.32 16.69,16.5 17.31,16.5 17.49,16.32 IC401.4 19.18,16.32 20.38,15.12 21.62,15.12 22.12,15.62 22.12,15.8 | 22.12,15.8 v22.12,16.25 | 22.12,15.8 22.3,16.16 v22.12,16.25 | 22.12,15.8 21.95,16.16 v22.12,16.25
  Bottom 0.203: IC201.14 26,17.88 26.12,17.75 26.12,17.12 25.75,16.75 | IC201.16 25,17.88 24.88,17.75 24.88,17.12 25.25,16.75 | R402.1 25.19,16 | 25.19,16 v25.5,15.69 25.5,16.12 | 25.25,16.75 25.5,16.5 | 25.5,16.5 25.5,16.12 | 25.75,16.75 25.5,16.5 | 25.25,16.75 25.75,16.75 | 25.19,16 25.38,16 25.5,16.12
USB.PRTCTL4-5  (via drill 0.3)
  Top 0.152: v21.25,19.5 21.25,19.18 | 21.25,19.18 21.25,19 20.88,18.62 20,18.62 19.38,19.25 16.38,19.25 15.44,18.32 | 15.44,18.32 v15.12,18 | 15.44,18.32 15.06,18.19 v15.12,18 | 15.44,18.32 15.31,17.94 v15.12,18 | 21.25,19.18 21.43,19.41 v21.25,19.5 | 21.25,19.18 21.07,19.41 v21.25,19.5
  Bottom 0.152: IC402.3 12.51,16.32 12.69,16.5 13.31,16.5 13.49,16.32 IC402.4 14.18,17.05 14.81,17.68 | R404.1 21.75,19 21.57,19.18 | 21.57,19.18 v21.25,19.5 | 14.81,17.68 v15.12,18 | 14.81,17.68 15.19,17.81 v15.12,18 | 14.81,17.68 14.94,18.06 v15.12,18 | 21.57,19.18 21.44,19.56 v21.25,19.5 | 21.57,19.18 21.19,19.31 v21.25,19.5
  Bottom 0.203: IC201.18 23.88,19.5 23.75,19.38 23.75,19.12 | IC201.17 23.88,19 | 23.88,19 23.62,19 | 23.62,19 R404.1 | 23.75,19.12 23.62,19 | 23.75,19.12 23.88,19
USB.VB_D  (via drill 0.3)
  Top 0.152: 27.42,16.46 27.34,16.52 | 55.94,18 55.93,18.01 55.93,21.18 54.56,22.55 51.97,22.55 48.92,25.6 46.33,25.6 39.62,18.9 35.81,18.9 34.29,17.37 31.85,17.37 30.94,16.46 27.42,16.46 | 55.94,18 v56.19,17.75 55.99,17.72 55.94,18 | 27.34,16.52 27.31,16.83 v27.12,16.75 | 27.34,16.52 27.08,16.55 v27.12,16.75 | 27.42,16.46 v27.12,16.75
  Top 0.254: C409.1 v52.62,7.44 | v56.19,17.75 56.88,17.75 TP6.TP
  Bottom 0.152: IC201.11 27.5,17.88 27.38,17.75 27.38,17.12 | 27.38,17.12 27.38,17 v27.12,16.75 | v56.19,17.75 55.87,17.43 | 55.87,17.43 55.02,16.58 55.02,11.73 53.03,9.75 53.03,7.85 52.94,7.76 | 52.94,7.76 v52.62,7.44 | 27.38,17.12 27.02,16.92 v27.12,16.75 | 27.38,17.12 27.32,16.73 v27.12,16.75 | 52.94,7.76 52.56,7.63 v52.62,7.44 | 52.94,7.76 52.81,7.37 v52.62,7.44 | 55.87,17.43 56.25,17.56 v56.19,17.75 | 55.87,17.43 56,17.81 v56.19,17.75
  Bottom 0.254: R410.1 R409.2 52.31,7.12 v52.62,7.44
VCC  (via drill 0.3)
  Bottom 0.254: R410.2 50.62,5.62 | 50.62,5.62 50.31,5.62 v50.31,5.81 | 50.62,5.62 50.5,5.75 | 50.62,5.62 50.5,5.5
  Bottom 0.406: TVS401.4 45.3,8.93 45.56,9.19 47.69,9.19 49.75,7.12 v49.75,6.38
  other vias: 49.75,5.81 50.31,5.25 49.75,5.25
  pour Bottom (rank 2, no thermals): 49.87,3.41 49.73,3.41 49.66,3.48 49.66,4.97 49.5,5.12 49.5,6.5 49.75,6.75 50,6.5 50,6.31 50.25,6.06 50.46,6.06 50.56,5.96 50.56,5.12 50.44,5 50.19,5 49.94,4.75 49.94,3.48
  pour Top (rank 2, no thermals): 51.75,5.12 51.75,5.78 51.65,5.88 50.75,5.88 50.56,6.06 50.25,6.06 50,6.31 50,6.53 49.9,6.62 49.6,6.62 49.5,6.53 49.5,5.1 49.6,5 50,5 51.5,3.5 51.5,2.91 51.6,2.81 52.4,2.81 52.5,2.91 52.5,4.59 52.4,4.69 52.19,4.69
VCCINT  (via drill 0.3)
  Top 0.254: C508.1 28.62,3.25 28.94,3.56 v28.94,3.75
  Top 0.381: v48.19,24.12 47.38,23.32 46.02,23.32 40.23,17.53 39.17,17.53 36.12,14.48 36.12,12.65 34.59,11.12 31.24,11.12 29.72,9.6 29.72,6.86 28.94,6.08 TP8.TP v28.94,3.75
  Bottom 0.254: IC502.5 27.88,3.38 28.25,3.75 v28.94,3.75
  Bottom 0.381: C519.1 49.42,24.8 48.75,24.12 v48.19,24.12
  pour Bottom (no thermals): 49.06,25.25 49.06,26.31 48.19,27.19 47.75,27.19 47.75,27.5 48.75,27.5 49.81,26.44 49.81,25.25
VDD18CORE  (via drill 0.3)
  Top 0.356: C205.1 v25.5,17.44
  Top 0.406: 27.5,27.81 v27.5,28.06 27.25,28.06 | 27.5,27.81 27.5,26 26.88,25.38 TP3.TP 26.88,19.88 26.38,19.38 25.88,19.38 25.5,19 C205.1 | C201.1 27.25,28.06 | 27.25,28.06 27.5,27.81
  Bottom 0.254: IC201.15 v25.5,17.44 | IC201.38 v27.5,28.06
  Bottom 0.356: C203.1 v27.5,28.06
VDD18ETHPLL  (via drill 0.3)
  Top 0.406: L201.1 C208.1 35.12,28.5 34.75,28.88 33.31,28.88 v32.5,28.06
  Bottom 0.254: IC201.48 v32.5,28.06
  Bottom 0.356: C210.1 v32.5,28.06
VDD18USBPLL  (via drill 0.3)
  Top 0.406: v34.12,19.88 34.05,19.95 C212.1 34.75,21 35.12,21.38 TP4.TP L201.2
  Bottom 0.254: IC201.62 34,20 v34.12,19.88
  Bottom 0.356: C213.1 34.19,19.81 v34.12,19.88
(copper drawn outside any net)
  shapes: VDD circle x1

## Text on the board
VDD: Moin!
tPlace: RPi 5V | Audio R / GPIO #18 | Audio GND | Audio L / GPIO #19 | OSHW | Speed | LAN | Duplex | PIOstack 1 | USB / 4+5 | luani.de | Link | SVN / $Rev: 447 $ | +5V In / GND | USB / Device | 01/16 | Run | USB / 2+3 | DM | DP
bPlace: PIOstack 1 | luani.de
Reference: DM, DP | PWR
